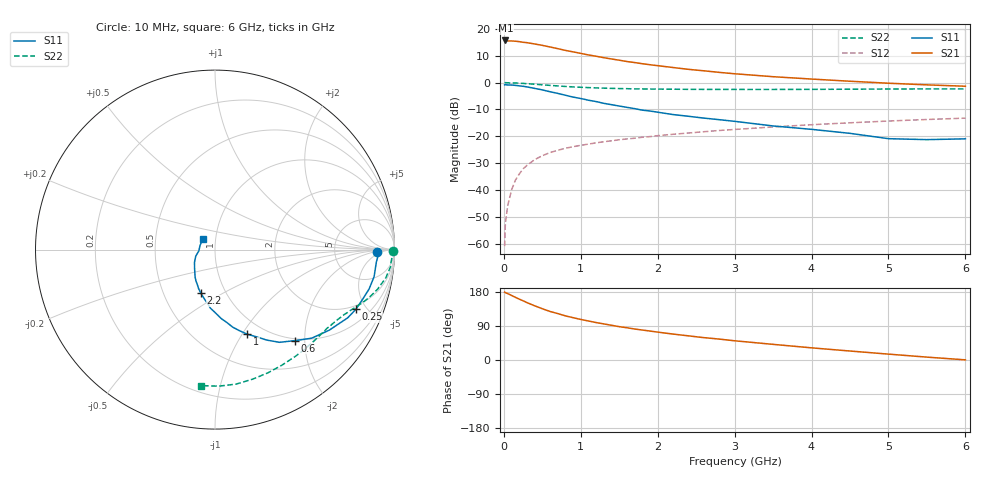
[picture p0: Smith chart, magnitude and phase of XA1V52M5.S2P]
! SIEMENS Discrete & RF Semiconductors
! BFY180
! Si NPN RF Bipolar Junction Transistor in MICRO-X
! VCE = 1.5 V  IC = 2.5 mA
! Common Emitter S-Parameters:  May  1997
# GHz  S  MA  R  50
!  f  S11  S21  S12  S22
! GHz  MAG  ANG  MAG  ANG  MAG  ANG  MAG  ANG
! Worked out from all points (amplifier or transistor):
!   36 points, 10 MHz to 6 GHz, reference 50 ohm
!   highest |S21| = 15.7 dB at 20 MHz (marker M1)
!   |S21| within 3 dB of that: start of sweep to 692.9 MHz
!   unconditionally stable (mu >= 1): 1.656 GHz to end of sweep
!   at 250 MHz: K = 0.20, MSG = 23.6 dB, |S12| = -32.1 dB
!   at 1.4 GHz: K = 0.92, MSG = 15.2 dB, |S12| = -21.7 dB
!   at 6 GHz: K = 1.15, MAG = 3.6 dB, |S12| = -13.2 dB
!   S11 on the Smith chart (normalised r, x): 10 MHz: 20, -3; 250 MHz: 1.74, -4.23; 600 MHz: 0.96, -1.80; 1 GHz: 0.83, -1.05; 2.2 GHz: 0.76, -0.39; 6 GHz: 0.87, +0.10
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0.01  0.9053 -0.9  5.954 179.1  0.0009 94.7  0.9892 -0.3
0.02  0.9109 -1.7  6.078 177.9  0.0024 84.0  0.9959 -0.8
0.05  0.9017 -4.4  5.962 175.3  0.0051 80.5  0.989 -1.9
0.1  0.8992 -9.6  5.948 170.4  0.01 85.5  0.9835 -3.9
0.2  0.869 -18.3  5.778 160.7  0.0198 78.9  0.9726 -7.6
0.25  0.8522 -23.0  5.622 156.3  0.0247 76.7  0.9651 -9.3
0.3  0.8314 -27.2  5.528 151.5  0.0287 73.7  0.9534 -10.8
0.4  0.7788 -35.2  5.231 143.1  0.0367 69.6  0.9313 -13.8
0.5  0.7305 -42.5  4.928 135.3  0.0435 65.2  0.907 -16.4
0.6  0.6751 -48.7  4.598 128.1  0.0497 62.6  0.8858 -18.6
0.8  0.581 -60.2  3.969 116.5  0.0598 57.4  0.8463 -22.3
1  0.505 -69.1  3.492 107.0  0.0679 54.0  0.8166 -25.5
1.1  0.469 -73.6  3.268 102.9  0.0715 53.0  0.8056 -26.7
1.3  0.4104 -80.9  2.902 95.2  0.0791 50.8  0.7869 -29.7
1.5  0.3656 -87.6  2.607 88.0  0.0861 49.2  0.7733 -32.5
1.8  0.3065 -97.2  2.242 79.1  0.0959 47.6  0.7604 -36.5
2.2  0.2537 -108.4  1.905 68.4  0.109 44.9  0.7515 -42.1
3  0.1897 -125.7  1.458 50.7  0.1339 39.7  0.7445 -53.1
3.5  0.1557 -136.9  1.286 41.3  0.1491 36.5  0.7441 -59.9
4.5  0.1134 -161.2  1.058 23.7  0.1782 28.8  0.7517 -73.8
5.5  0.0866 164.6  0.906 7.6  0.2054 20.8  0.7613 -88.4
6  0.0896 139.4  0.854 0.4  0.2176 16.5  0.7616 -95.8
